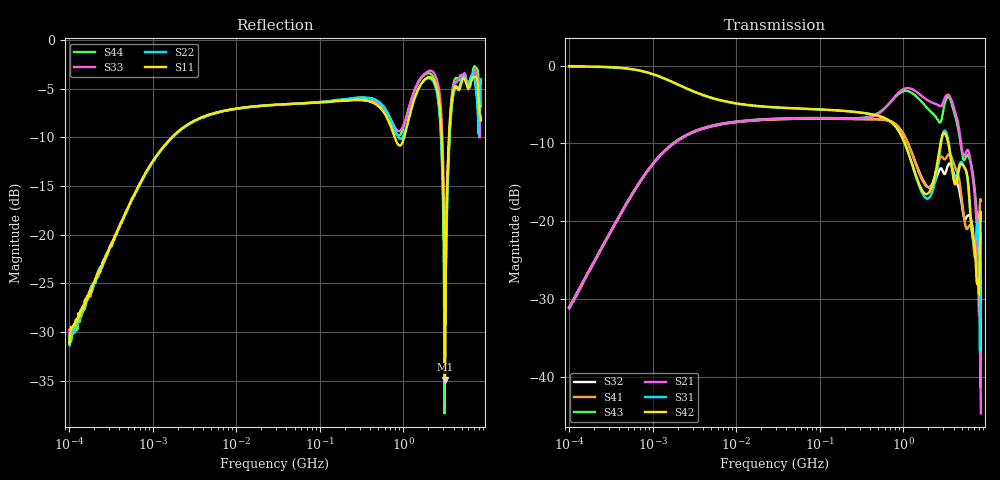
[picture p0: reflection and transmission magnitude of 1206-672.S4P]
!Agilent Technologies,E5071C,MY46110495,A.10.06
!Date: Tue Jun 06 12:36:57 2017
!Data & Calibration Information:
!Freq	S11:SOLT4(ON)	S12:SOLT4(ON)	S13:SOLT4(ON)	S14:SOLT4(ON)
!	S21:SOLT4(ON)	S22:SOLT4(ON)	S23:SOLT4(ON)	S24:SOLT4(ON)
!	S31:SOLT4(ON)	S32:SOLT4(ON)	S33:SOLT4(ON)	S34:SOLT4(ON)
!	S41:SOLT4(ON)	S42:SOLT4(ON)	S43:SOLT4(ON)	S44:SOLT4(ON)
!PortZ  Port1:50+j0  Port2:50+j0  Port3:50+j0  Port4:50+j0
!Above PortZ is port z conversion or system Z0 setting when saving the data.
!When reading, reference impedance value at option line is always used.
# Hz S dB R 50
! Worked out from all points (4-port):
!   801 points, 100 kHz to 8.5 GHz, reference 50 ohm
!   strongest paths, dB at 100 kHz, 1.721 MHz, 29.51 MHz, 502.3 MHz, 8.5 GHz:
!     S42: -0.1, -2.1, -5.4, -6.5, -18.8
!     S31: -0.1, -2.1, -5.4, -6.4, -21.5
!     S21: -31.2, -10.1, -6.8, -6.2, -44.6
!     S43: -31.1, -10.1, -6.8, -6.1, -30.7
!     S41: -31.1, -10.1, -6.9, -6.9, -17.4
!     S32: -31.0, -10.1, -6.9, -6.9, -25.5
!   lowest |S11| = -34.9 dB at 3.155 GHz (marker M1), VSWR 1.04, Z = 51.6 + j0.945 ohm
!   |S11| at or under -10 dB: start of sweep to 1.694 MHz; 790.6 MHz to 1.025 GHz (234.3 MHz wide, 25.8 % of centre); 2.886 GHz to 3.535 GHz (649.6 MHz wide, 20.2 % of centre)
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100000  -31.00 69.1  -31.13 86.4  -0.13 -1.4  -31.10 -94.6
        -31.17 85.9  -31.12 70.8  -31.27 -95.2  -0.11 -1.4
        -0.14 -1.4  -31.03 -94.2  -29.77 75.8  -30.96 85.8
        -31.07 -94.0  -0.08 -1.6  -31.09 85.7  -30.30 75.3
8898533  -7.11 12.5  -7.28 12.4  -4.78 -10.2  -7.32 -168.9
         -7.28 12.4  -7.12 12.7  -7.33 -168.8  -4.78 -10.2
         -4.79 -10.2  -7.33 -168.8  -7.11 12.6  -7.27 12.4
         -7.30 -168.9  -4.77 -10.3  -7.26 12.5  -7.12 12.7
2.134648e9  -3.82 69.1  -4.68 -16.3  -16.69 170.6  -15.47 39.1
            -4.69 -16.3  -3.96 67.1  -15.67 34.1  -15.91 163.2
            -16.69 170.8  -15.67 34.2  -3.13 64.0  -5.95 -18.1
            -15.46 39.2  -15.92 163.2  -5.92 -18.1  -3.45 63.6
3.154505e9  -34.90 30.6  -4.13 -18.7  -8.34 82.4  -12.07 1.1
            -4.14 -18.7  -24.57 113.0  -13.90 -2.3  -8.74 70.7
            -8.36 82.5  -13.91 -2.4  -22.99 -12.0  -4.78 -7.7
            -12.05 1.4  -8.74 70.8  -4.76 -7.7  -30.98 -163.2
5.236375e9  -3.93 -79.2  -11.48 -53.1  -12.78 7.8  -18.79 -147.5
            -11.49 -53.0  -3.76 -79.4  -19.10 -164.9  -12.84 5.5
            -12.80 7.8  -19.11 -164.9  -3.53 -82.5  -12.02 -43.2
            -18.81 -147.0  -12.84 5.5  -12.02 -43.1  -3.55 -79.1
6.842542e9  -3.87 17.0  -14.65 -80.4  -22.37 -14.7  -22.59 38.4
            -14.64 -80.2  -3.55 10.0  -21.43 41.2  -22.09 -27.3
            -22.38 -14.4  -21.41 41.4  -3.69 14.5  -14.01 -57.9
            -22.61 38.9  -22.07 -27.0  -13.98 -57.7  -3.08 21.3
8.5e9  -8.24 111.6  -44.15 -163.0  -21.44 50.4  -17.37 29.7
       -44.64 -164.3  -4.03 121.9  -25.51 76.6  -18.80 28.2
       -21.46 50.6  -25.54 76.7  -4.19 125.9  -30.77 55.1
       -17.36 30.3  -18.79 28.6  -30.66 55.2  -6.82 97.6
